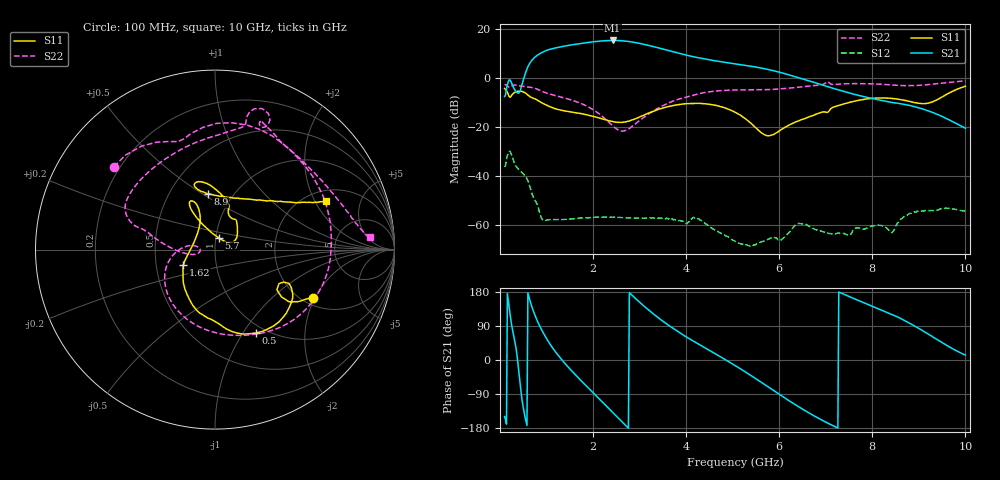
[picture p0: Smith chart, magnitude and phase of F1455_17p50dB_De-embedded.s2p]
! Integrated Device Technology
! Corporate Headquarters
! 6024 Silver Creek Valley Road
! San Jose, CA 95138  USA
! Phone:  1-408-284-8200
! Toll Free:  1-800-223-1366
! Webpage:  http://www.idt.com/
! Timing and RF Division
! 515 Groton Road, Suite 102
! Westford, MA 01886-6024
! Device:  F1455
! Description: 6-bit 0.5 dB Transmit Variable Gain Amplifier
! Frequency:  1400.0 -  2300.00 MHz
! Package:  6x6 mm Thin QFN Plastic Package: 28 pin
! State:  35
! Atten State:  17.5 dB
! Voltage:  +5.00 Volts
! Current:  217.623 mA
! Data:  The device was measured on a the F1455 evaluation board which has
!  individual transmission lines to the RF pins.  Data was collected
!  using a calibrated network analyzer.  The evaluation board was
!  de-embedded using a TRL calibration technique.
!  The reference plane is the edge of the package pin.
!  Pin  1 = CSb
!  Pin  2 = DATA
!  Pin  3 = CLK
!  Pin  4 = RSET
!  Pin  5 = GND
!  Pin  6 = RFIN  = Port 1
!  Pin  7 = GND
!  Pin  8 = NC
!  Pin  9 = NC
!  Pin 10 = NC
!  Pin 11 = NC
!  Pin 12 = NC
!  Pin 13 = NC
!  Pin 14 = /STBY
!  Pin 15 = GND
!  Pin 16 = RFOUT  = Port 2
!  Pin 17 = GND
!  Pin 18 = NC
!  Pin 19 = NC
!  Pin 20 = NC
!  Pin 21 = GND
!  Pin 22 = NC
!  Pin 23 = GND
!  Pin 24 = NC
!  Pin 25 = NC
!  Pin 26 = NC
!  Pin 27 = GND
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# GHz S dB R 50
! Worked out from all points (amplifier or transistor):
!   496 points, 100 MHz to 10 GHz, reference 50 ohm
!   highest |S21| = 15.2 dB at 2.42 GHz (marker M1)
!   |S21| within 3 dB of that: 1.205 GHz to 3.4 GHz (2.194 GHz wide, 95.3 % of centre)
!   unconditionally stable (mu >= 1): start of sweep to end of sweep
!   at 1.74 GHz: K = 62.23, MAG = 14.6 dB, |S12| = -57.0 dB
!   at 5.06 GHz: K = 360.82, MAG = 7.5 dB, |S12| = -66.6 dB
!   at 10 GHz: K = 373.93, MAG = -11.9 dB, |S12| = -54.2 dB
!   S11 on the Smith chart (normalised r, x): 100 MHz: 2.25, -1.92; 500 MHz: 0.90, -1.14; 1.62 GHz: 0.69, -0.12; 5.7 GHz: 1.03, +0.14; 8.9 GHz: 0.76, +0.53; 10 GHz: 2.48, +2.48
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0.1  -4.34 -26.3  -7.60 -149.2  -36.31 46.7  -2.76 140.7
0.26  -6.87 -24.6  -2.55 86.2  -31.97 -76.6  -3.30 95.6
0.38  -5.48 -41.5  -6.21 -1.7  -36.81 -116.0  -3.09 57.7
0.5  -5.73 -63.8  -1.00 -125.1  -39.09 -154.1  -3.44 27.3
0.68  -8.00 -90.7  6.99 142.6  -46.67 141.2  -3.93 -14.0
0.82  -9.25 -108.9  9.41 98.4  -52.71 115.9  -4.76 -45.3
0.96  -10.78 -123.3  10.84 65.3  -58.14 126.1  -5.92 -70.6
1.28  -13.07 -143.1  12.52 8.0  -57.72 99.8  -7.68 -114.3
1.62  -14.14 -154.0  13.66 -39.0  -57.30 71.6  -9.55 -147.1
1.76  -14.62 -157.8  14.06 -56.6  -57.02 61.9  -10.57 -158.1
2.1  -16.19 -168.9  14.87 -98.4  -56.67 41.9  -14.24 179.1
2.42  -17.82 171.1  15.21 -138.0  -56.78 26.9  -19.49 169.7
2.8  -17.40 135.8  14.71 175.4  -57.04 12.5  -20.32 -167.6
3.1  -15.11 118.3  13.60 141.6  -57.15 4.8  -15.99 -172.1
3.4  -12.89 112.3  12.21 111.7  -57.04 -5.8  -12.34 178.0
4.1  -10.42 115.7  8.82 53.9  -57.42 -21.1  -7.39 164.1
5.06  -14.06 119.4  5.69 -15.1  -66.56 -54.7  -4.94 148.9
5.7  -23.28 72.0  3.66 -65.9  -66.08 -25.0  -4.84 122.7
6.7  -15.51 42.0  -1.56 -144.0  -61.03 -127.8  -3.23 78.8
8.36  -8.28 107.0  -9.80 123.3  -62.12 127.0  -2.82 62.8
8.9  -10.07 97.5  -11.77 90.2  -54.54 128.8  -3.16 41.3
10  -3.40 23.7  -20.52 13.2  -54.20 48.5  -1.27 4.7
